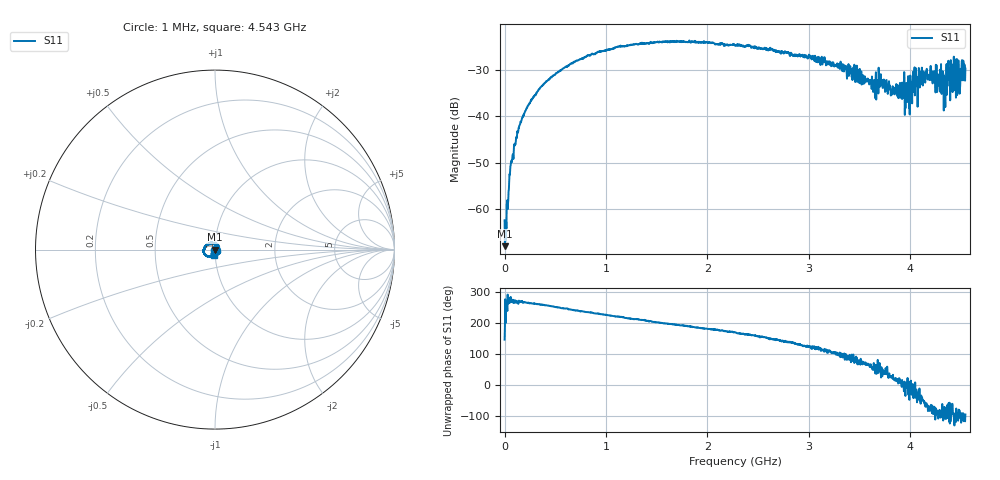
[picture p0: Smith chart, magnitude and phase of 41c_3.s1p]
# HZ S RI R 50
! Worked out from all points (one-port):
!   1515 points, 1 MHz to 4.543 GHz, reference 50 ohm
!   lowest |S11| = -68.1 dB at 4 MHz (marker M1), VSWR 1.00, Z = 50 - j0.00574 ohm
!   |S11| at or under -10 dB: start of sweep to end of sweep
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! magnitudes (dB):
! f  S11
! 1 MHz  -62.5
! 4 MHz  -68.1
! 25 MHz  -59.4
! 43 MHz  -55.8
! 76 MHz  -49.1
! 160 MHz  -41.2
! 340 MHz  -34.1
! 571 MHz  -29.8
! 1.138 GHz  -24.8
! 1.705 GHz  -23.9
! 2.272 GHz  -24.7
! 2.842 GHz  -26.9
! 3.409 GHz  -29.2
! 3.652 GHz  -36.0
! 3.703 GHz  -31.6
! 3.829 GHz  -34.1
! 3.976 GHz  -34.4
! 4.009 GHz  -34.5
! 4.045 GHz  -35.5
! 4.147 GHz  -32.7
! 4.219 GHz  -32.9
! 4.33 GHz  -38.8
! 4.351 GHz  -35.4
! 4.378 GHz  -30.5
! 4.405 GHz  -32.9
! 4.447 GHz  -31.4
! 4.471 GHz  -34.4
! 4.543 GHz  -29.7
